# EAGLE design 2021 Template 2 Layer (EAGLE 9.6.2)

## Sheet 1 of 2: Template
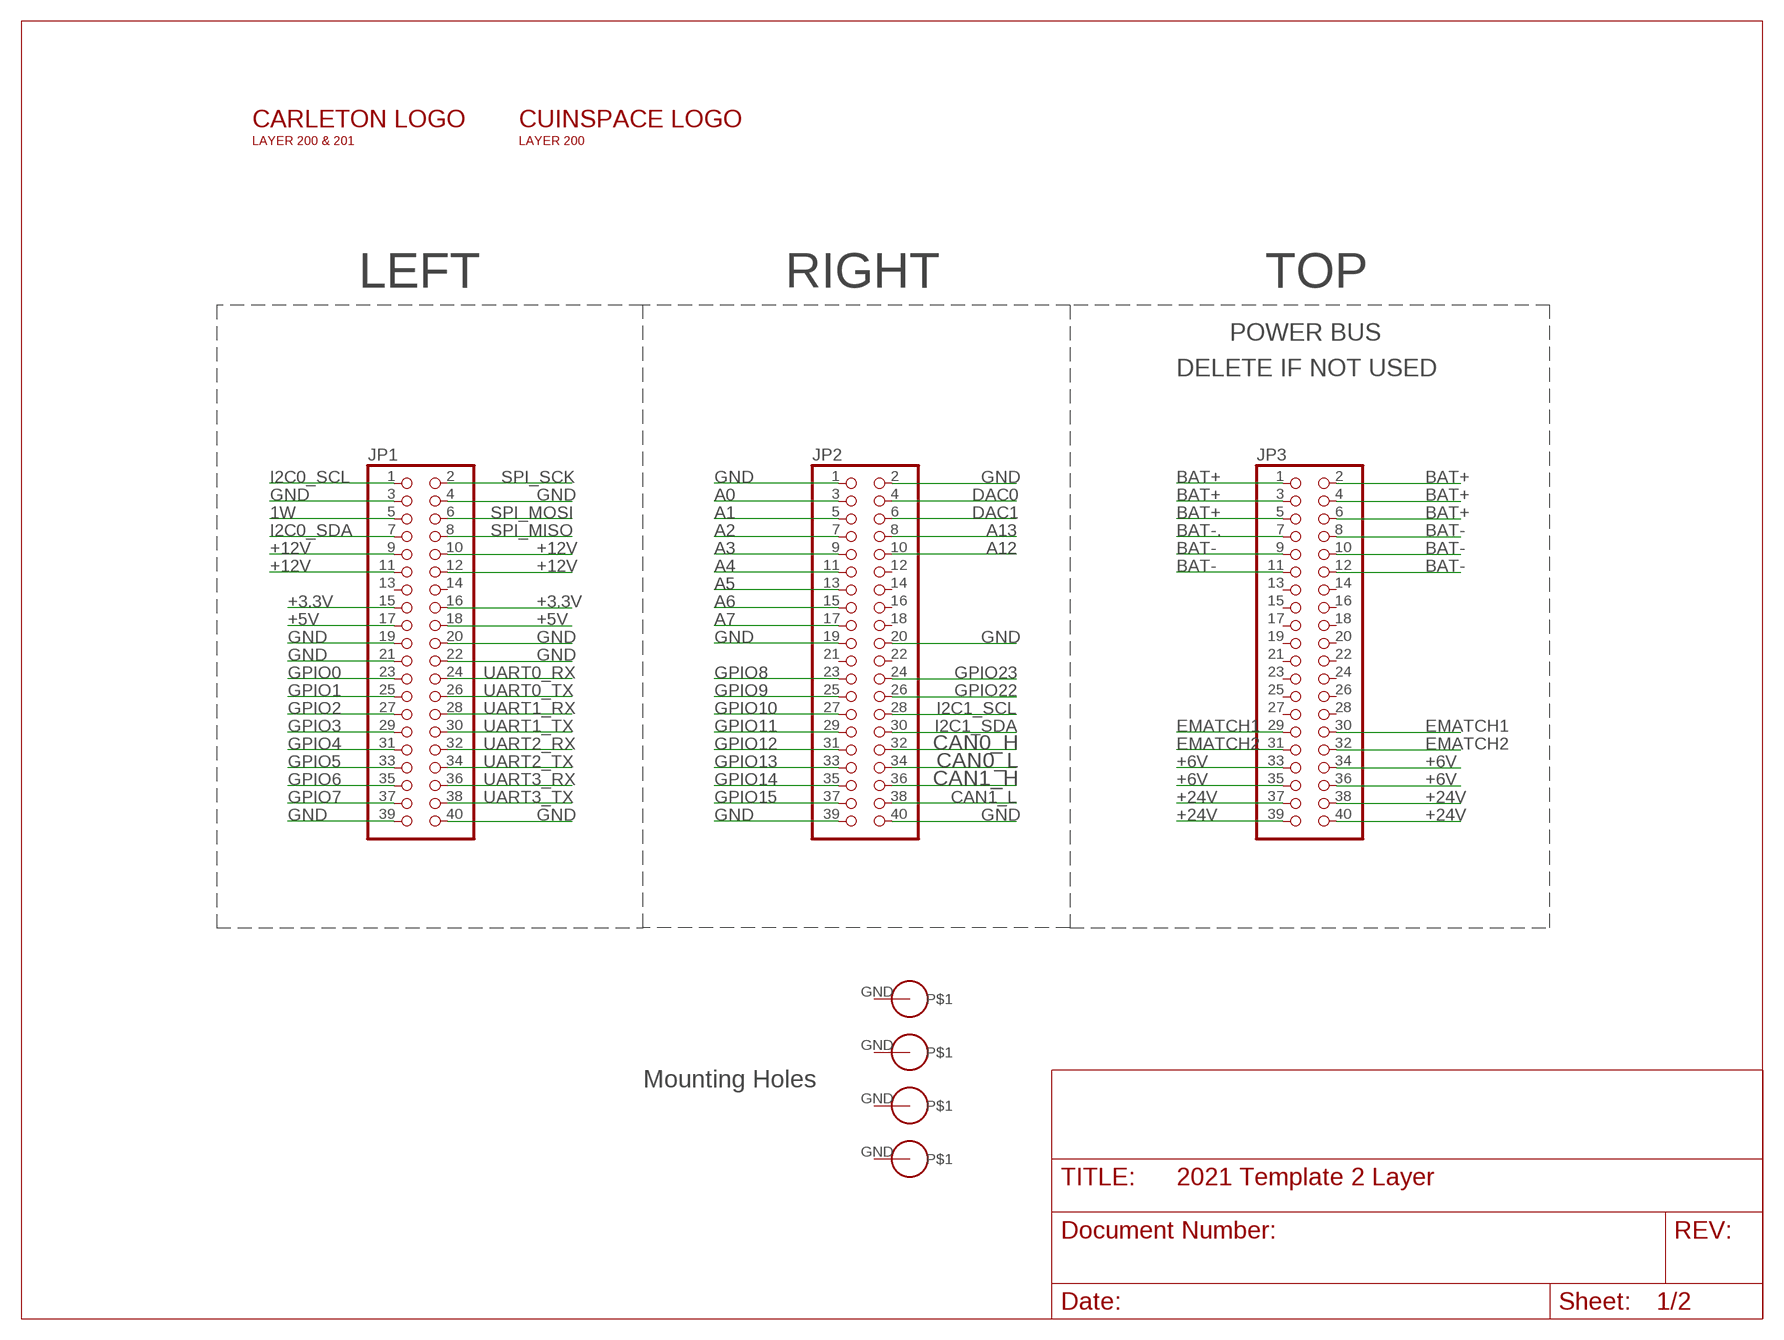
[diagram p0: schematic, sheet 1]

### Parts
$$U$1  PS/104-MOUNTING-HOLE  [PC/104-MOUNTING-HOLE]
JP1  PINHD-2X20  [2X20]
JP2  PINHD-2X20  [2X20]
JP3  PINHD-2X20  [2X20]
U$1  PS/104-MOUNTING-HOLE  [PC/104-MOUNTING-HOLE]
U$2  PS/104-MOUNTING-HOLE  [PC/104-MOUNTING-HOLE]
U$3  PS/104-MOUNTING-HOLE  [PC/104-MOUNTING-HOLE]
U$4  CARLETON3CM  [CARLETONU_3CM]
U$6  INSPACE3CM_L  [INSPACE_3CM_LETTERS]

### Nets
1W: JP1.5
+3.3V: JP1.15 JP1.16
+5V: JP1.17 JP1.18
+6V: JP3.33 JP3.34 JP3.35 JP3.36
+12V: JP1.9 JP1.10 JP1.11 JP1.12
+24V: JP3.37 JP3.38 JP3.39 JP3.40
A0: JP2.3
A1: JP2.5
A2: JP2.7
A3: JP2.9
A4: JP2.11
A5: JP2.13
A6: JP2.15
A7: JP2.17
A12: JP2.10
A13: JP2.8
BAT+: JP3.1 JP3.2 JP3.3 JP3.4 JP3.5 JP3.6
BAT-: JP3.8 JP3.9 JP3.10 JP3.11 JP3.12
BAT-.: JP3.7
CAN0_H: JP2.32
CAN0_L: JP2.34
CAN1_H: JP2.36
CAN1_L: JP2.38
DAC0: JP2.4
DAC1: JP2.6
EMATCH1: JP3.29 JP3.30
EMATCH2: JP3.31 JP3.32
GND [New Class]: JP1.3 JP1.4 JP1.19 JP1.20 JP1.21 JP1.22 JP1.39 JP1.40 JP2.1 JP2.2 JP2.19 JP2.20 JP2.39 JP2.40
GPIO0: JP1.23
GPIO1: JP1.25
GPIO2: JP1.27
GPIO3: JP1.29
GPIO4: JP1.31
GPIO5: JP1.33
GPIO6: JP1.35
GPIO7: JP1.37
GPIO8: JP2.23
GPIO9: JP2.25
GPIO10: JP2.27
GPIO11: JP2.29
GPIO12: JP2.31
GPIO13: JP2.33
GPIO14: JP2.35
GPIO15: JP2.37
GPIO22: JP2.26
GPIO23: JP2.24
I2C0_SCL: JP1.1
I2C0_SDA: JP1.7
I2C1_SCL: JP2.28
I2C1_SDA: JP2.30
SPI_MISO: JP1.8
SPI_MOSI: JP1.6
SPI_SCK: JP1.2
UART0_RX: JP1.24
UART0_TX: JP1.26
UART1_RX: JP1.28
UART1_TX: JP1.30
UART2_RX: JP1.32
UART2_TX: JP1.34
UART3_RX: JP1.36
UART3_TX: JP1.38
Unconnected: $$U$1.GND JP1.13 JP1.14 JP2.12 JP2.14 JP2.16 JP2.18 JP2.21 JP2.22 JP3.13 JP3.14 JP3.15 JP3.16 JP3.17 JP3.18 JP3.19 JP3.20 JP3.21 JP3.22 JP3.23 JP3.24 JP3.25 JP3.26 JP3.27 JP3.28 U$1.GND U$2.GND U$3.GND

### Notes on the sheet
- LEFT | RIGHT | TOP
- POWER BUS
- DELETE IF NOT USED
- Mounting Holes

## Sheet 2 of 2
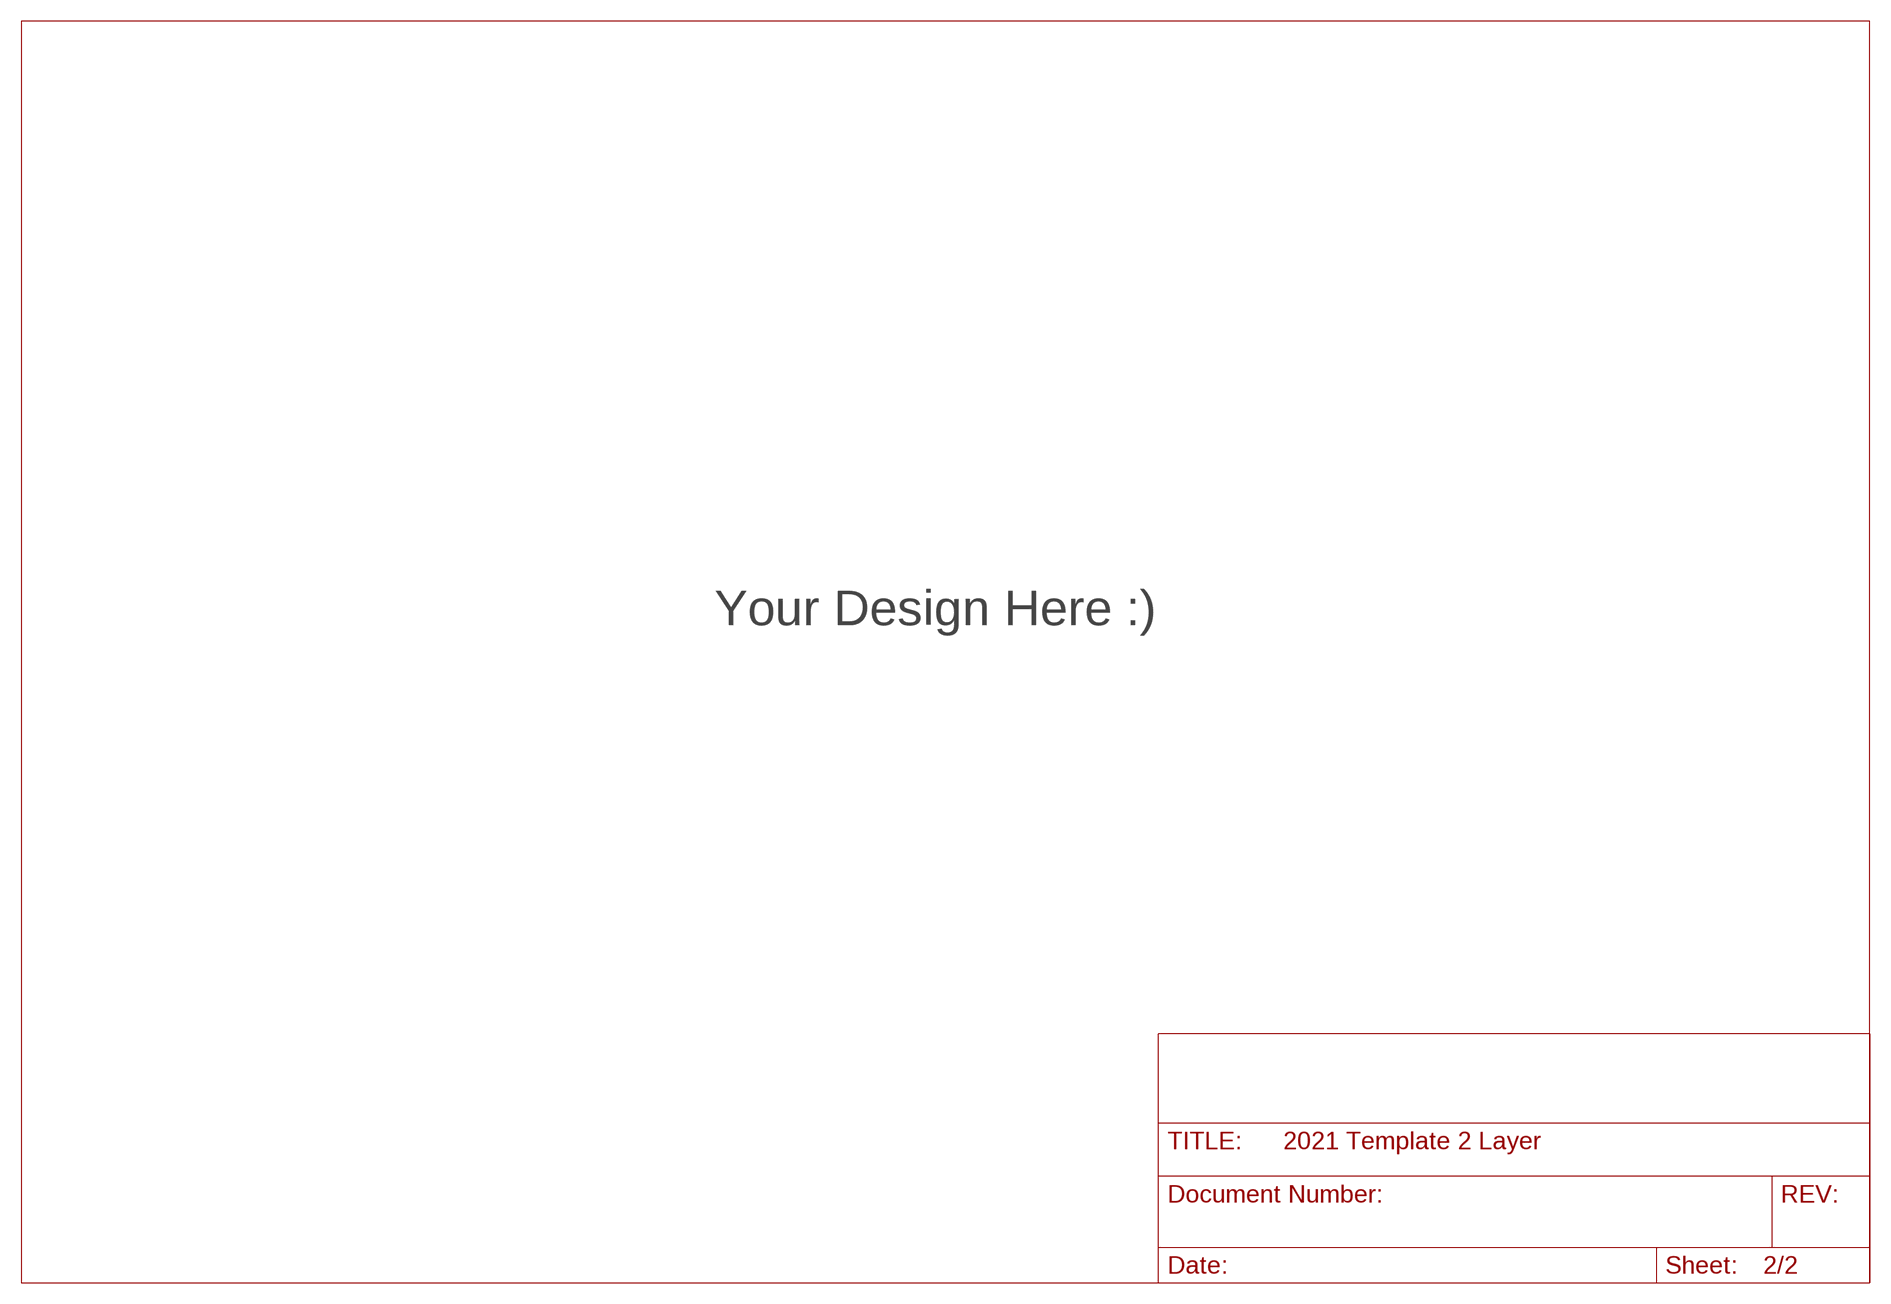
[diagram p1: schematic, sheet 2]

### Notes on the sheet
- Your Design Here :)

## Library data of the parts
$$U$1 U$1-U$3 = CU inSpace 2019 Parts:PS/104-MOUNTING-HOLE: Mounting hole for PC/104 board.
JP1-JP3 = pinhead:PINHD-2X20: PIN HEADER
U$4 = Logos:CARLETON
U$6 = Logos:INSPACE

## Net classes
2 diff pairs: width 0.254 mm

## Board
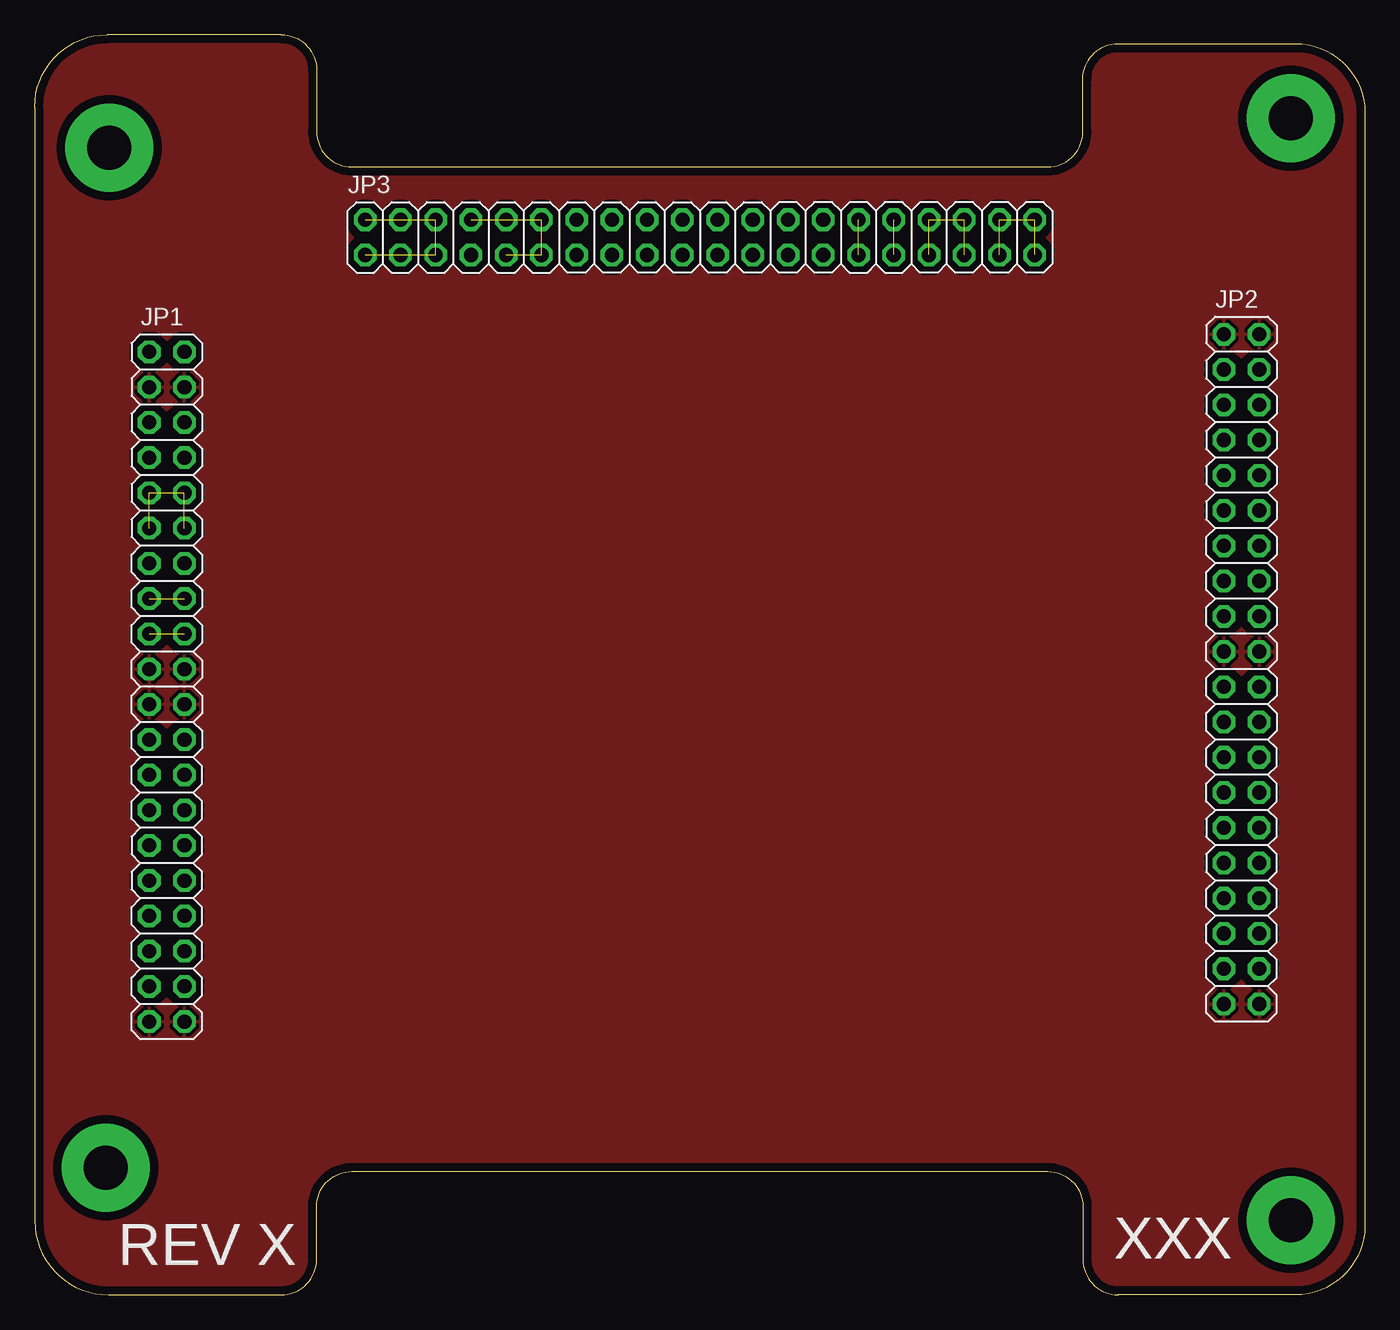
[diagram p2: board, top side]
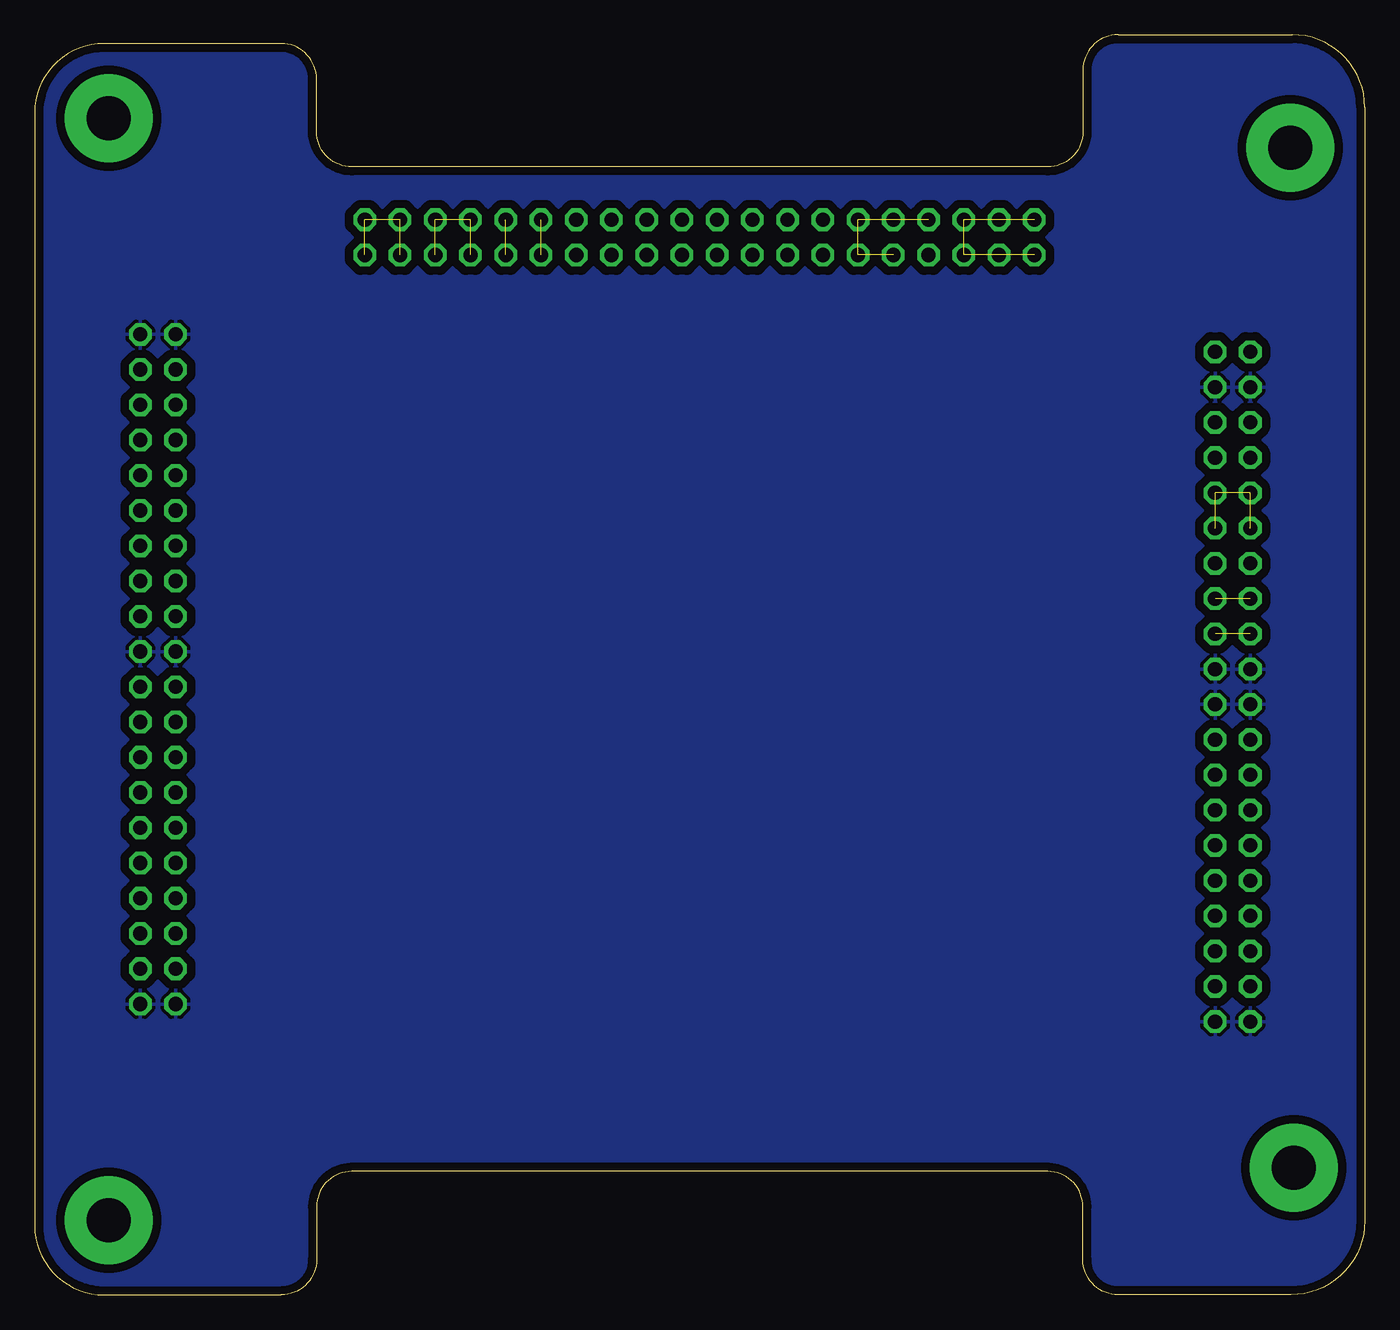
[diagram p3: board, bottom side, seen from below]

Size 95.89 x 90.81 mm. Coordinates in mm from the lower left corner, seen from the top.
Outline: 0,85.57 0,5.33 arc90 5.33,0 17.78,0 arc90 20.32,2.54 20.32,6.35 arc-90 22.86,8.89 73.03,8.89 arc-90 75.56,6.35 75.56,2.54 arc90 78.11,0 90.89,0 arc90 95.89,5 95.89,85.17 arc90 90.89,90.17 78.11,90.17 arc90 75.56,87.63 75.56,83.82 arc-90 73.03,81.28 22.86,81.28 arc-90 20.32,83.82 20.32,88.27 arc90 17.78,90.81 5.23,90.81 arc90 0,85.57
Copper layers (1*16): Top 0.035mm / dielectric 1.53mm / Bottom 0.035mm
Design rules "JLC 2 Layer": minimum track width 5mil, minimum drill 0.2mm, track to track 3.5mil, track to pad 3.5mil, pad to pad 5mil, via to via 10mil, smd to smd 0mil, copper to edge 10mil, drill to drill 10mil, minimum pad ring 12mil, minimum via ring 5mil, stop-mask expansion 4mil, vias tented up to drill 0mil, thermal gap 10mil

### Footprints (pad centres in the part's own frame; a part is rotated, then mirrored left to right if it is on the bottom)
PC/104-MOUNTING-HOLE = drill 3.175 pad 6.35: GND 0,0
2X20 = drill 1.016 octagon: 1 -24.13,-1.27; 2 -24.13,1.27; 3 -21.59,-1.27; 4 -21.59,1.27; 5 -19.05,-1.27; 6 -19.05,1.27; 7 -16.51,-1.27; 8 -16.51,1.27; 9 -13.97,-1.27; 10 -13.97,1.27; 11 -11.43,-1.27; 12 -11.43,1.27; 13 -8.89,-1.27; 14 -8.89,1.27; 15 -6.35,-1.27; 16 -6.35,1.27; 17 -3.81,-1.27; 18 -3.81,1.27; 19 -1.27,-1.27; 20 -1.27,1.27; 21 1.27,-1.27; 22 1.27,1.27; 23 3.81,-1.27; 24 3.81,1.27; 25 6.35,-1.27; 26 6.35,1.27; 27 8.89,-1.27; 28 8.89,1.27; 29 11.43,-1.27; 30 11.43,1.27; 31 13.97,-1.27; 32 13.97,1.27; 33 16.51,-1.27; 34 16.51,1.27; 35 19.05,-1.27; 36 19.05,1.27; 37 21.59,-1.27; 38 21.59,1.27; 39 24.13,-1.27; 40 24.13,1.27

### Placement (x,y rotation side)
$$U$1  5.13,9.17 0 top
JP1  9.53,43.81 270 top
JP2  87,45.09 270 top
JP3  47.96,76.2 0 top
U$1  90.55,84.79 0 top
U$2  5.36,82.65 0 top
U$3  90.55,5.36 0 top
U$4  not placed on the board
U$6  not placed on the board

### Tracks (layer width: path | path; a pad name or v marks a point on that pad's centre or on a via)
+3.3V  (1 unrouted)
+5V  (1 unrouted)
+6V  (3 unrouted)
+12V  (3 unrouted)
+24V  (3 unrouted)
BAT+  (5 unrouted)
BAT-  (4 unrouted)
EMATCH1  (1 unrouted)
EMATCH2  (1 unrouted)
GND
  pour Top (isolate 0.61): 0,0 0,90.81 93.98,90.81 95.89,90.81 95.89,0
  pour Top (isolate 0.61): 0,0 0,90.81 93.98,90.81 95.89,90.81 95.89,0
  pour Bottom (isolate 0.61): 0,0 0,90.81 93.98,90.81 95.89,90.81 95.89,0

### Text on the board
tPlace: YOUR NAME
tNames: XXX | REV X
